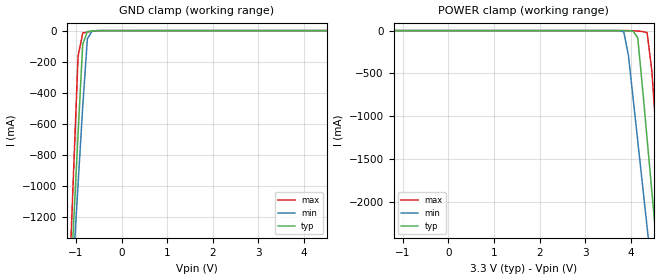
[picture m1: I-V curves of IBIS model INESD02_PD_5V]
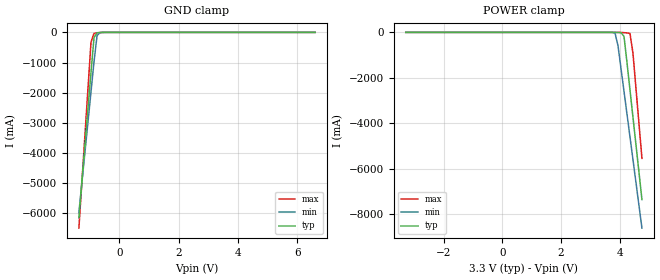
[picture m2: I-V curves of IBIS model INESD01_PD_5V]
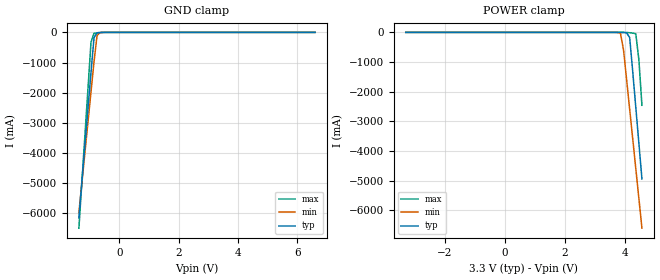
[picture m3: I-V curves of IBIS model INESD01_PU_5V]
|   This file is an IBIS representation of the   |
|   Integrated Device Technology, Inc.   |
|   ICS8538-31   |
|   LOW SKEW, 1-TO-8, CRYSTAL OSCILLATOR/LVCMOS-TO-3.3V LVPECL FANOUT BUFFER |
[IBIS Ver]   4.1
[File name]   8538_31_3v3.ibs
[File Rev]   1.0
[Date]   27 May 2010
[Source]   Originated at Integrated Device Technology, Inc.
[Disclaimer]
IDT hereby grants the user of this IBIS model a non-exclusive,
nontransferable license to use this IBIS model under the following terms.
Before using this IBIS model, the user should read this license.
If the user does not accept these terms,  the IBIS model should be
returned to IDT within 30 days.
   The user is granted this license only to use the IBIS model and
is not granted rights to sell, load, rent, lease or license the IBIS
model in whole or in part, or in modified form to anyone other than
user. User may modify the IBIS model to suit its specific
applications but rights to derivative works and such modifications
shall belong to IDT.
   This IBIS model is provided on an "AS IS" basis and IDT makes
absolutely no warranty with respect to the information contained
herein. IDT DISCLAIMS AND CUSTOMER WAIVES ALL WARRANTIES, EXPRESS
OR IMPLIED, INCLUDING WARRANTIES OF MERCHANTABILITY OR FITNESS FOR
A PARTICULAR PURPOSE. The entire risk as to quality and performance
is with the Customer. ACCORDINGLY, IN NO EVENT SHALL THE COMPANY BE
LIABLE FOR ANY DAMAGES, WHETHER IN CONTRACT OR TORT,INCLUDING ANY
LOST PROFITS OR OTHER INCIDENTAL, CONSEQUENTIAL, EXEMPLARY, OR
PUNITIVE DAMAGES ARISING OUT OF THE USE OR APPLICATION OF THE IBIS
model provided in this package. Further, IDT reserves the right to
make changes without notice to any product herein to improve
reliability, function, or design. IDT does not convey any license
under patent rights or any other intellectual property rights,
including those of third parties.
   IDT is not obligated to provide maintenance or support
for the licensed IBIS model.
[Copyright]   Copyright 2010 by Integrated Device Technology, Inc.
[Component]   841602GI
[Manufacturer] Integrated Device Technology, Inc.
[Package]
|TSSOP 28 Lead
|   typ   min   max
R_pkg   60.65m   52.4m   68.9m
L_pkg   1.989nH   1.431nH   2.547nH
C_pkg   0.314pF   0.254pF   0.374pF
[Pin]   signal_name   model_name   R_pin   L_pin   C_pin
1   CLK   INESD02_PD_5V   68.9m   2.547n   0.374p
2   CLK_SEL   INESD01_PD_5V   66.2m   2.360n   0.254p
3   CLK_EN   INESD01_PU_5V   63.4m   2.174n   0.334p
4   VEE   GND   60.6m   1.988n   0.314p
5   nQ7   ONF01_PECL01ALT_   57.9m   1.802n   0.294p
6   Q7   ONF01_PECL01ALT_   55.1m   1.616n   0.274p
7   VCCO   POWER   52.4m   1.431n   0.254p
8   nQ6   ONF01_PECL01ALT_   52.4m   1.431n   0.254p
9   Q6   ONF01_PECL01ALT_   55.1m   1.616n   0.274p
10   nQ5   ONF01_PECL01ALT_   57.9m   1.802n   0.294p
11   Q5   ONF01_PECL01ALT_   60.6m   1.988n   0.314p
12   VEE   GND   63.4m   2.174n   0.334p
13   nQ4   ONF01_PECL01ALT_   66.2m   2.360n   0.254p
14   Q4   ONF01_PECL01ALT_   68.9m   2.547n   0.374p
15   nQ3   ONF01_PECL01ALT_   68.9m   2.547n   0.374p
16   Q3   ONF01_PECL01ALT_   66.2m   2.360n   0.254p
17   VCCO   POWER   63.4m   2.174n   0.334p
18   nQ2   ONF01_PECL01ALT_   60.6m   1.988n   0.314p
19   Q2   ONF01_PECL01ALT_   57.9m   1.802n   0.294p
20   nQ1   ONF01_PECL01ALT_   55.1m   1.616n   0.274p
21   Q1   ONF01_PECL01ALT_   52.4m   1.431n   0.254p
22   VCCO   POWER   52.4m   1.431n   0.254p
23   nQ0   ONF01_PECL01ALT_   55.1m   1.616n   0.274p
24   Q0   ONF01_PECL01ALT_   57.9m   1.802n   0.294p
25   VEE   GND   60.6m   1.988n   0.314p
26   XTAL_OUT   NC   63.4m   2.174n   0.334p
27   XTAL_IN   NC   66.2m   2.360n   0.254p
28   VCC   POWER   68.9m   2.547n   0.374p
[Diff Pin]  inv_pin  vdiff tdelay_typ tdelay_min  tdelay_max
24   23   NA   0   0   0
21   20   NA   0   0   0
19   18   NA   0   0   0
16   15   NA   0   0   0
14   13   NA   0   0   0
11   10   NA   0   0   0
9   8   NA   0   0   0
6   5   NA   0   0   0
| Models and submodels in the file (4): INESD02_PD_5V (Input), INESD01_PD_5V (Input), INESD01_PU_5V (Input), ONF01_PECL01ALT_ (Output_ECL)
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[Model]   INESD02_PD_5V
Model_type  Input
Polarity   Non-Inverting
Vinl = 0.8V
Vinh = 2.0V
|   typ   min   max
C_comp   2pF   1.5pF   2.5pF
|   typ   min   max
[Voltage range]  3.3V   3.135V   3.465V
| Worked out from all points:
|   GND clamp passes 1 mA (typ) near -0.58 V on its own axis
[GND_clamp]
|Voltage   I(typ)   I(min)   I(max)
-1.973V   -6.688A    -6A        -7.863A
-1.157V   -1.867A    -1.988A    -1.704A
-1.055V   -1.265A    -1.488A    -934.1mA
-952.6mV  -663.4mA   -987.4mA   -164.5mA
-850.5mV  -87.6mA    -487.5mA   -16.04mA
-748.5mV  -6.317mA   -52.72mA   -9.171mA
-646.4mV  -1.91mA    -2.66mA    -4.148mA
-340.2mV  -9.776uA   -8.593uA   -12.08uA
6.6V      128.6uA    131.6uA    121.8uA
[POWER_clamp]
|Voltage   I(typ)   I(min)   I(max)
-3.3V     128.6uA    128.3uA    124.8uA
3.64V     -9.776uA   -103.4uA   -3.241uA
3.844V    -417.5uA   -15.85mA   -26.94uA
3.946V    -1.91mA    -296.1mA   -290.3uA
4.048V    -6.317mA   -795.7mA   -1.934mA
4.151V    -87.6mA    -1.296A    -5.908mA
4.355V    -1.265A    -2.297A    -23.83mA
4.457V    -1.867A    -2.799A    -459.4mA
4.559V    -2.47A     -3.3A      -1.229A
4.661V    -3.072A    -3.801A    -1.999A
4.763V    -3.675A    -4.303A    -2.769A
5.681V    -9.099A    -8.82A     -9.698A
[Model]   INESD01_PD_5V
Model_type  Input
Polarity   Non-Inverting
Vinl = 0.8V
Vinh = 2.0V
|   typ   min   max
C_comp   2pF   1.5pF   2.5pF
|   typ   min   max
[Voltage range]  3.3V   3.135V   3.465V
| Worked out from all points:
|   GND clamp passes 1 mA (typ) near -0.55 V on its own axis
[GND_clamp]
|Voltage   I(typ)   I(min)   I(max)
-1.361V   -6.144A    -5.981A    -6.488A
-952.6mV  -1.327A    -1.975A    -329.1mA
-850.5mV  -175.2mA   -975mA     -32.08mA
-748.5mV  -12.63mA   -105.4mA   -18.35mA
-646.4mV  -3.815mA   -5.31mA    -8.297mA
6.6V      128.6uA    131.6uA    121.8uA
[POWER_clamp]
|Voltage   I(typ)   I(min)   I(max)
-3.3V     128.6uA    128.3uA    124.8uA
3.64V     -12.95uA   -197.2uA   -3.249uA
3.844V    -826.8uA   -31.68mA   -47.07uA
3.946V    -3.815mA   -592.1mA   -573.6uA
4.048V    -12.63mA   -1.591A    -3.867mA
4.151V    -175.2mA   -2.592A    -11.82mA
4.253V    -1.327A    -3.593A    -22.84mA
4.355V    -2.53A     -4.595A    -47.66mA
4.457V    -3.735A    -5.597A    -918.8mA
4.763V    -7.349A    -8.606A    -5.538A
[Model]   INESD01_PU_5V
Model_type  Input
Polarity   Non-Inverting
Vinl = 0.8V
Vinh = 2.0V
|   typ   min   max
C_comp   2pF   1.5pF   2.5pF
|   typ   min   max
[Voltage range]  3.3V   3.135V   3.465V
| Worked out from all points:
|   GND clamp passes 1 mA (typ) near -0.55 V on its own axis
[GND_clamp]
|Voltage   I(typ)   I(min)   I(max)
-1.361V   -6.144A    -5.981A    -6.488A
-952.6mV  -1.327A    -1.975A    -329.1mA
-850.5mV  -175.3mA   -975.1mA   -32.14mA
-748.5mV  -12.69mA   -105.5mA   -18.41mA
-646.4mV  -3.879mA   -5.373mA   -8.361mA
6.6V      64.3uA     69.07uA    57.85uA
[POWER_clamp]
|Voltage   I(typ)   I(min)   I(max)
-3.3V     64.3uA     65.78uA    60.89uA
3.64V     -77.24uA   -259.7uA   -67.18uA
3.844V    -891.1uA   -31.75mA   -111uA
3.946V    -3.879mA   -592.2mA   -637.6uA
4.048V    -12.69mA   -1.591A    -3.93mA
4.151V    -175.3mA   -2.592A    -11.88mA
4.253V    -1.327A    -3.593A    -22.9mA
4.355V    -2.53A     -4.595A    -47.73mA
4.457V    -3.735A    -5.597A    -918.9mA
4.559V    -4.939A    -6.6A      -2.458A
